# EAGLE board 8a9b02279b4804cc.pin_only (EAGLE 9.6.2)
REV: C

Size 17.78 x 20.7 mm. Coordinates in mm from the lower left corner, seen from the top.
Outline: 17.78,18.16 17.78,2.54 arc-90 15.24,0 2.54,0 arc-90 0,2.54 0,18.16 arc-90 2.54,20.7 15.24,20.7 arc-90 17.78,18.16
Copper layers (1*16): Top 0.035mm / dielectric 1.5mm / Bottom 0.035mm
Design rules "adafruit 6-6": minimum track width 6mil, minimum drill 15.5mil, track to track 6mil, track to pad 6mil, pad to pad 6mil, via to via 6mil, smd to smd 6mil, copper to edge 10mil, drill to drill 8mil, minimum pad ring 10mil, minimum via ring 8mil, stop-mask expansion 2mil, vias tented up to drill 20mil, thermal gap 10mil
Net classes: 1 power: width 0.254 mm; 2 gnd: width 0.254 mm

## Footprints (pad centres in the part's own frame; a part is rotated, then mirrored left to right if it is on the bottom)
_0805MP = smd 1.2 x 1.3: 1 -1.016,0; 2 1.016,0
_0402NO = smd 0.6 x 0.6: 1 -0.508,0; 2 0.508,0
JST_SH4_SKINNY = smd 0.5 x 1.55: 1 -1.5,2.514; 2 -0.5,2.514; 3 0.5,2.514; 4 1.5,2.514 | smd 1.2 x 1.8: MT1 -2.8,-1.386; MT2 2.8,-1.386
SOD-323_MINI = smd 0.9 x 0.8: A 1.07,0; C -1.07,0
QFN32_5MM = smd 0.8 x 0.25: 1 -2.5,1.75; 2 -2.5,1.25; 3 -2.5,0.75; 4 -2.5,0.25; 5 -2.5,-0.25; 6 -2.5,-0.75; 7 -2.5,-1.25; 8 -2.5,-1.75; 17 2.5,-1.75; 18 2.5,-1.25; 19 2.5,-0.75; 20 2.5,-0.25; 21 2.5,0.25; 22 2.5,0.75; 23 2.5,1.25; 24 2.5,1.75 | smd 0.25 x 0.8: 9 -1.75,-2.5; 10 -1.25,-2.5; 11 -0.75,-2.5; 12 -0.25,-2.5; 13 0.25,-2.5; 14 0.75,-2.5; 15 1.25,-2.5; 16 1.75,-2.5; 25 1.75,2.5; 26 1.25,2.5; 27 0.75,2.5; 28 0.25,2.5; 29 -0.25,2.5; 30 -0.75,2.5; 31 -1.25,2.5; 32 -1.75,2.5 | smd 3.5 x 3.5: 33 0,0
1X07_CASTEL = drill 1 pad 1.778: 1 -7.62,0; 2 -5.08,0; 3 -2.54,0; 4 0,0; 5 2.54,0; 6 5.08,0; 7 7.62,0 | drill 1 pad 1.778 long: 1C -7.62,-1.27; 2C -5.08,-1.27; 3C -2.54,-1.27; 4C 0,-1.27; 5C 2.54,-1.27; 6C 5.08,-1.27; 7C 7.62,-1.27
SK6805_1515 = smd 0.5 x 0.5: 1 -0.5,-0.45; 2 0.5,-0.45; 3 0.5,0.45; 4 -0.5,0.45
BTN_KMR2_4.6X2.8 = smd 0.9 x 0.9: A 2.05,0.8; A' -2.05,0.8; B 2.05,-0.8; B' -2.05,-0.8
B1,27 = smd 1.27 x 1.27: TP 0,0
TESTPOINT_RECT_1X3MM = smd 3 x 1.5: P$1 0,0
SOT23-5 = smd 0.55 x 1.2: 1 -0.95,-1.3; 2 0,-1.3; 3 0.95,-1.3; 4 0.95,1.3; 5 -0.95,1.3
SOIC8_150MIL = smd 0.6 x 2.2: 1 -1.905,-2.6; 2 -0.635,-2.6; 3 0.635,-2.6; 4 1.905,-2.6; 5 1.905,2.6; 6 0.635,2.6; 7 -0.635,2.6; 8 -1.905,2.6
FIDUCIAL_1MM = smd 1 x 1: 1 0,0
USB_C_CUSB31-CFM2AX-01-X = smd 0.575 x 1.15: A1B12 -3.2,3.545; A4B9 -2.4,3.545; B1A12 3.2,3.545; B4A9 2.4,3.545 | smd 0.275 x 1.15: A5 -1.25,3.545; A6 -0.25,3.545; A7 0.25,3.545; A8 1.25,3.545; B5 1.75,3.545; B6 0.75,3.545; B7 -0.75,3.545; B8 -1.75,3.545 | drill 0.6 pad 1 long: M1 -4.32,2.97; M2 4.32,2.97; M3 -4.32,-1.21; M4 4.32,-1.21 | hole 0.65: 2.89,2.47; -2.89,2.47

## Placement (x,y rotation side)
C1  10uF  [_0805MP]  13.69,10.73 270 top
C2  1uF  [_0402NO]  4.95,12.97 180 top
C3  1uF  [_0402NO]  7.71,12.98 0 top
C8  10uF  [_0805MP]  13.64,7.09 270 top
CONN1  STEMMA_I2C_QTSKINNY  [JST_SH4_SKINNY]  7.01,2.39 0 top
D1  NSR0320  [SOD-323_MINI]  11.71,12.95 180 top
IC3  ATSAMD21E  [QFN32_5MM]  6.53,9.15 0 top
JP1  [1X07_CASTEL]  1.27,10.35 270 top
JP3  [1X07_CASTEL]  16.51,10.35 90 top
LED1  WS2812B_SK6805_1515  [SK6805_1515]  10.87,6.97 270 top
Q2  reset  [BTN_KMR2_4.6X2.8]  12.57,2.79 90 top
R1  5.1K  [_0402NO]  4.27,5.14 0 top
R5  5.1K  [_0402NO]  3.43,16.6 0 top
R6  5.1K  [_0402NO]  14.35,17.04 180 top
SWC  TPB1,27  [B1,27]  10.16,15.24 0 bottom
SWC1  TPB1,27  [B1,27]  8.89,12.95 0 bottom
SWD  TPB1,27  [B1,27]  7.62,15.24 0 bottom
TP1  [TESTPOINT_RECT_1X3MM]  10.79,18.92 270 bottom
TP2  [TESTPOINT_RECT_1X3MM]  6.99,18.92 270 bottom
U1  AP2112K-3.3  [SOT23-5]  11.43,10.21 180 top
U2  [SOIC8_150MIL]  7.18,9.39 90 bottom
U$6  FIDUCIAL_1MM  [FIDUCIAL_1MM]  5.89,1.52 0 top
U$8  FIDUCIAL_1MM  [FIDUCIAL_1MM]  8.89,19.68 0 top
U$11  [QTPY_BOT]  17.78,0 0 bottom
U$12  [PCBFEAT-REV-040]  8.89,19.41 0 bottom
U$13  [QTPY_TOP]  0,0 0 top
X6  USB TYPE C  [USB_C_CUSB31-CFM2AX-01-X]  8.89,17.91 180 top

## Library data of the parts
C1-C3 C8 CONN1 D1 JP1 JP3 LED1 Q2 R1 R5 R6 TP1 TP2 U2 U$12 X6 = microbuilder
IC3 = adafruit_micro
SWC SWC1 SWD = testpad
U1 = adafruit_power
U$6 U$8 = microbuilder; BOM: EXCLUDE
U$11 U$13 = itsy_silks

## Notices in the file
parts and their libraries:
microbuilder: This work is placed in the public domain, and may be freely used for commercial and non-commercial work with the following conditions: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
